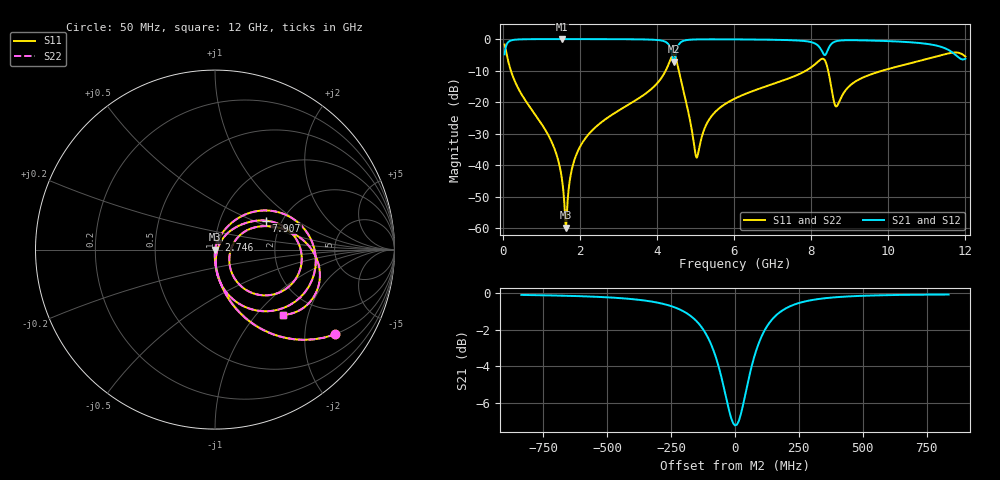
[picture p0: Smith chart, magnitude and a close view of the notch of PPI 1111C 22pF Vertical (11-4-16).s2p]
# GHz S MA R 50
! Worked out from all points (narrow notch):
!   1601 points, 50 MHz to 12 GHz, reference 50 ohm
!   highest |S21| = -0.01 dB at 1.529 GHz (marker M1); lowest = -7.2 dB at 4.442 GHz (marker M2)
!   notch at M2: 7.0 dB deep, 140 MHz wide at half that depth
!   lowest |S11| = -59.8 dB at 1.641 GHz (marker M3), VSWR 1.00, Z = 50.1 - j0.00402 ohm
!   |S11| at or under -10 dB: 212.1 MHz to 4.228 GHz (4.016 GHz wide, 181 % of centre); 4.567 GHz to 7.867 GHz (3.3 GHz wide, 53.1 % of centre); 8.441 GHz to 9.852 GHz (1.411 GHz wide, 15.4 % of centre)
!   |S22| runs from -59.8 to -1.7 dB; largest |S21 - S12| = 0
!   S11 on the Smith chart (normalised r, x): 50 MHz: 0.99, -2.85; 2.746 GHz: 1.03, +0.11; 7.907 GHz: 1.66, +0.60; 12 GHz: 1.40, -1.40
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0.05  0.8205 -35.1  0.5715 54.9  0.5715 54.9  0.8205 -35.1
0.2964688  0.2285 -78.1  0.973 11.8  0.973 11.8  0.2285 -78.1
1.245  0.02529 -92.6  0.9987 -4.6  0.9987 -4.6  0.02529 -92.6
1.528812  0.006522 -88.3  0.9989 -7.0  0.9989 -7.0  0.006522 -88.3
1.640844  0.001026 -2.2  0.9989 -7.9  0.9989 -7.9  0.001026 -2.2
1.812625  0.009617 74.3  0.9988 -9.3  0.9988 -9.3  0.009617 74.3
2.044156  0.02164 75.8  0.9985 -11.1  0.9985 -11.1  0.02164 75.8
2.746219  0.05811 71.9  0.9966 -16.5  0.9966 -16.5  0.05811 71.9
4.038312  0.2095 54.5  0.9626 -31.3  0.9626 -31.3  0.2095 54.5
4.307188  0.4055 31.2  0.8133 -43.6  0.8133 -43.6  0.4055 31.2
4.441625  0.5667 -17.5  0.4356 -25.9  0.4356 -25.9  0.5667 -17.5
4.635813  0.2061 -79.1  0.9043 -11.0  0.9043 -11.0  0.2061 -79.1
5.031656  0.01325 -15.3  0.9866 -24.0  0.9866 -24.0  0.01325 -15.3
5.382688  0.05627 53.9  0.9908 -28.7  0.9908 -28.7  0.05627 53.9
6.025  0.1143 52.6  0.9881 -34.9  0.9881 -34.9  0.1143 52.6
7.907125  0.327 29.6  0.9177 -55.6  0.9177 -55.6  0.327 29.6
8.019156  0.3637 24.8  0.888 -58.3  0.888 -58.3  0.3637 24.8
8.347781  0.4668 -24.6  0.5577 -50.1  0.5577 -50.1  0.4668 -24.6
8.661469  0.08606 -6.4  0.9289 -42.8  0.9289 -42.8  0.08606 -6.4
10.01331  0.3373 22.6  0.9274 -65.1  0.9274 -65.1  0.3373 22.6
11.58175  0.5966 -11.9  0.6617 -86.8  0.6617 -86.8  0.5966 -11.9
12  0.5246 -43.9  0.4892 -63.3  0.4892 -63.3  0.5246 -43.9
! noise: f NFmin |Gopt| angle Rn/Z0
0.05  0.0003505  0.8599  1.192  0.0005356
1.372  0.003513  0.6555  6.706  0.001937
2.701  0.006377  0.6341  12.64  0.003242
4.031  0.0236  0.8364  19.03  0.02967
5.36  0.01919  0.7492  25.22  0.01469
6.682  0.01773  0.6818  30.57  0.01006
8.012  0.05725  0.8717  36.85  0.0866
9.341  0.03491  0.7739  42.18  0.02752
10.67  0.04721  0.8111  47.44  0.04378
12  0.3074  0.9656  53.23  1.619
